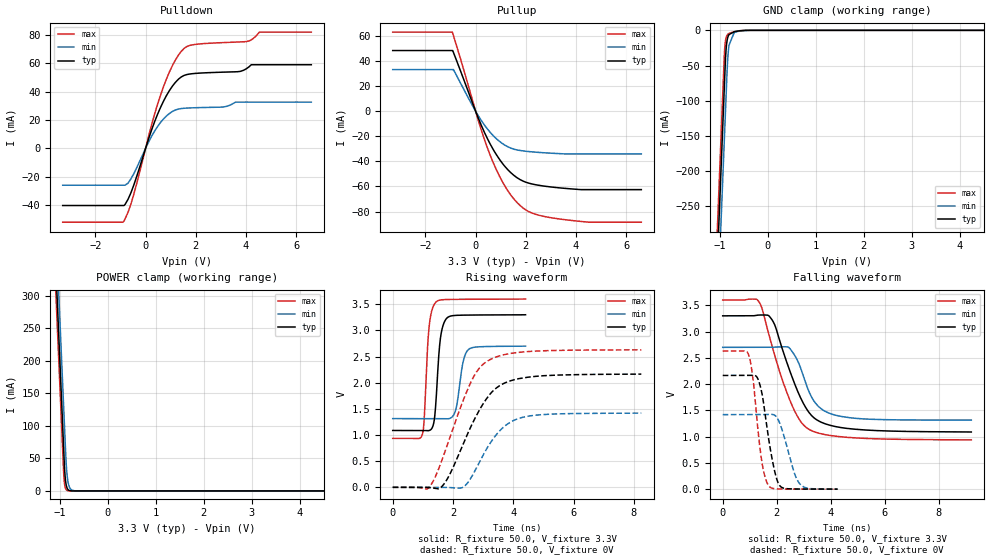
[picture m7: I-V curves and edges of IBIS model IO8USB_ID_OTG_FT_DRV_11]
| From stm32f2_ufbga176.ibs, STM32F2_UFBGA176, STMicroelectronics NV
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| *** New cell (Generated with 5.14beta1 (Sep 20 2010 13:23:23))
[Model]   IO8USB_ID_OTG_FT_DRV_11
Model_type 3-state
Polarity   Non-Inverting
Enable   Active-Low
| CAP_THRESHOLD on pad IOV33 is "CMOS" :
| Rising=10.0% of vddio   Falling=90.0% of vddio
| C_comp min and max val. don't necessarily correlate with the min and max pvt
| but are the smallest and greatest pad capacitance found.
| var   typ   min   max
C_comp   2.14880pF  2.04280pF  2.27520pF
Vmeas = 1.65V   | Reference voltage for timing measurements
Cref  = 50.0pF   | Timing specification test load capacitance value
Rref  = 10.0MOhm   | Timing specification test load resistance value
Vref  = 1.65V   | Timing specification test load voltage
[Model Spec]
| variable   typ   min   max
[Temperature Range] 25.0 125.0 -40.0
| variable   typ   min   max
[Voltage Range] 3.3V 2.7V 3.6V
| variable   typ   min   max
[POWER Clamp Reference] 3.3V 2.7V 3.6V
| variable   typ   min   max
[GND Clamp Reference] 0V 0V 0V
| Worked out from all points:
|   slope of the pulldown table from 0 to 0.495 V, typ, clamps not added: 20 ohm
|   slope of the pullup table from 0 to 0.495 V, typ, clamps not added: 21.7 ohm
|   GND clamp passes 1 mA (typ) near -0.62 V on its own axis
|   POWER clamp passes 1 mA (typ) near -0.81 V on its own axis
|   rising waveform, R_fixture 50.0, V_fixture 3.3V: 20-80 % time 164ps typ, 213ps min, 147ps max; typ from 1.09 V to 3.3 V
|   falling waveform, R_fixture 50.0, V_fixture 3.3V: 20-80 % time 1.01ns typ, 719ps min, 1.03ns max; typ from 3.3 V to 1.09 V
|   rising waveform, R_fixture 50.0, V_fixture 0V: 20-80 % time 1.11ns typ, 947ps min, 1.04ns max; typ from 0 V to 2.16 V
|   falling waveform, R_fixture 50.0, V_fixture 0V: 20-80 % time 399ps typ, 474ps min, 328ps max; typ from 2.17 V to 0 V
[POWER Clamp]
-3.3V     4.11A      4.173A     4.072A
-1.09V    352.5mA    415.9mA    314.5mA
-1.05V    284.5mA    347.9mA    246.5mA
-1.01V    216.5mA    279.9mA    178.5mA
-920mV    63.51mA    126.9mA    25.85mA
-900mV    31.51mA    92.9mA     9.552mA
-890mV    21.35mA    75.9mA     5.807mA
-870mV    9.804mA    44.01mA    2.146mA
-840mV    3.05mA     18.36mA    482.1uA
-780mV    295.2uA    3.194mA    24.34uA
-660mV    2.764uA    96.54uA    62.42nA
6.6V      0A         0A         0A
[GND Clamp]
-3.3V     -4.149A    -4.223A    -4.103A
-1.06V    -340.6mA   -415.4mA   -294.6mA
-940mV    -136.6mA   -211.4mA   -90.55mA
-910mV    -85.56mA   -160.4mA   -39.55mA
-900mV    -68.56mA   -143.4mA   -26.56mA
-880mV    -36.74mA   -109.4mA   -13.48mA
-860mV    -19.55mA   -75.41mA   -8.247mA
-840mV    -11.31mA   -44.9mA    -5.968mA
-810mV    -6.021mA   -21.14mA   -4.415mA
-700mV    -1.968mA   -2.918mA   -1.891mA
-470mV    -106.7uA   -266.5uA   -47.83uA
6.6V      9.456nA    1.186uA    63.86pA
| variable   typ   min   max
[Pullup Reference] 3.3V 2.7V 3.6V
| variable   typ   min   max
[Pulldown Reference] 0V 0V 0V
[Pullup]
-3.3V     48.28mA    33.11mA    63.01mA
-930mV    48.28mA    33.11mA    63.01mA
-880mV    46.73mA    33.11mA    60.08mA
120mV     -6.142mA   -4.065mA   -8.189mA
590mV     -26.5mA    -17.07mA   -35.52mA
1.18V     -44.36mA   -27.27mA   -60.11mA
1.54V     -51.43mA   -30.39mA   -70.35mA
1.89V     -55.75mA   -31.69mA   -77.18mA
2.48V     -58.98mA   -32.83mA   -82.75mA
3.6V      -61.62mA   -34.07mA   -86.61mA
4.51V     -62.54mA   -34.07mA   -88.51mA
6.6V      -62.54mA   -34.07mA   -88.51mA
[Pulldown]
-3.3V     -40.25mA   -25.94mA   -51.99mA
-870mV    -40.25mA   -25.94mA   -51.33mA
-700mV    -35.92mA   -24.51mA   -45.06mA
-470mV    -25.89mA   -17.87mA   -32.39mA
240mV     12.97mA    8.52mA     16.62mA
590mV     28.62mA    18.11mA    37.2mA
1.07V     43.85mA    26mA       58.31mA
1.54V     51.42mA    28.24mA    70.48mA
2.01V     52.82mA    28.63mA    73.27mA
4.01V     56.01mA    32.56mA    75.18mA
4.53V     58.9mA     32.56mA    81.88mA
6.6V      58.9mA     32.56mA    81.88mA
[Ramp]
dV/dt_r 1.29886V/1.11508ns 851.3068mV/947.60324ps 1.57728V/1.0365ns
dV/dt_f 1.3277V/1.00896ns 831.60271mV/719.74296ps 1.59819V/1.03442ns
R_load = 50.0
| Removed startup time: 0s 0s 0s  .
| Removed end time: 4.404ns.
[Rising Waveform]
R_fixture   = 50.0
V_fixture   = 3.3V
V_fixture_min = 2.7V
V_fixture_max = 3.6V
0s        1.087V     1.314V     936.3mV
981ps     1.087V     1.314V     1.006V
1.043ns   1.086V     1.314V     1.295V
1.206ns   1.086V     1.314V     3.061V
1.431ns   1.615V     1.314V     3.541V
1.582ns   2.847V     1.313V     3.583V
1.794ns   3.235V     1.309V     3.591V
2.084ns   3.288V     1.471V     3.594V
2.51ns    3.294V     2.634V     3.596V
4.406ns   3.3V       2.7V       3.6V
| Removed startup time: 0s 0s 0s  .
| Removed end time: 9.196ns.
[Falling Waveform]
R_fixture   = 50.0
V_fixture   = 3.3V
V_fixture_min = 2.7V
V_fixture_max = 3.6V
0s        3.3V       2.7V       3.6V
1.353ns   3.315V     2.7V       3.557V
1.681ns   3.31V      2.7V       2.997V
1.862ns   3.193V     2.702V     2.659V
2.453ns   2.294V     2.695V     1.734V
2.796ns   1.836V     2.417V     1.36V
3.216ns   1.445V     1.829V     1.132V
3.679ns   1.267V     1.517V     1.05V
4.427ns   1.169V     1.381V     994.5mV
9.198ns   1.089V     1.314V     937.8mV
| Removed startup time: 0s 0s 0s  .
| Removed end time: 8.242ns.
[Rising Waveform]
R_fixture   = 50.0
V_fixture   = 0V
V_fixture_min = 0V
V_fixture_max = 0V
0s        7.752nV    280.7nV    5.712nV
1.23ns    -5.807mV   3.61uV     15.89mV
1.524ns   -27.76mV   112.5uV    353.5mV
1.703ns   65.14mV    292.3uV    632.6mV
2.355ns   853.1mV    9.979mV    1.688V
2.753ns   1.348V     344.9mV    2.184V
3.224ns   1.78V      836.7mV    2.442V
3.717ns   1.996V     1.171V     2.539V
4.397ns   2.099V     1.35V      2.592V
8.244ns   2.164V     1.418V     2.629V
| Removed startup time: 0s 0s 0s  .
| Removed end time: 4.246ns.
[Falling Waveform]
R_fixture   = 50.0
V_fixture   = 0V
V_fixture_min = 0V
V_fixture_max = 0V
0s        2.165V     1.419V     2.629V
966ps     2.166V     1.419V     2.546V
1.142ns   2.17V      1.419V     2.014V
1.357ns   2.022V     1.418V     876.9mV
1.513ns   1.634V     1.42V      339.9mV
1.711ns   920.3mV    1.424V     57.18mV
1.943ns   296.8mV    1.4V       7.517mV
2.152ns   44.4mV     1.198V     2.977mV
2.846ns   2.156mV    105.1mV    1.058mV
4.248ns   93.15uV    36.11uV    94.57uV
